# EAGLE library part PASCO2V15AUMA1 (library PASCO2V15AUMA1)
Air Quality Sensors ENVIRONMENTAL SENSING,Carbon Dioxide (CO2) Sensor I2C, PWM, UART Source: Datasheet
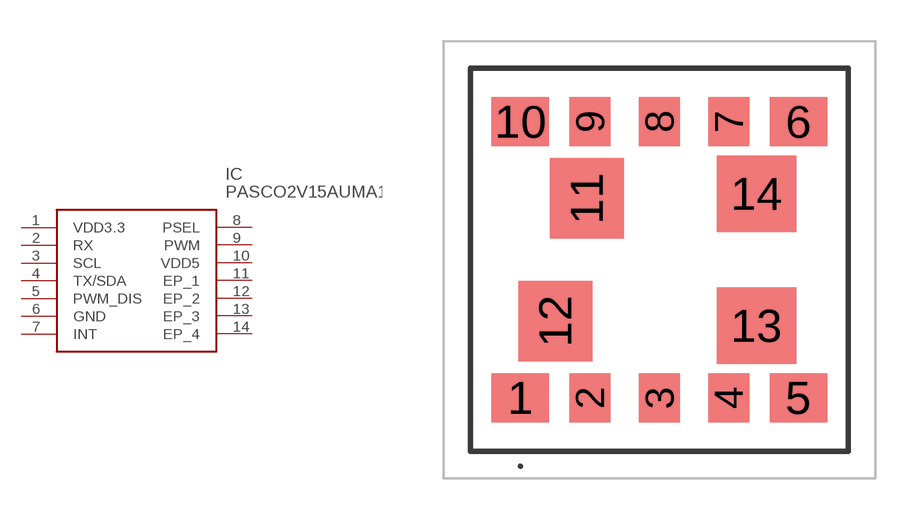
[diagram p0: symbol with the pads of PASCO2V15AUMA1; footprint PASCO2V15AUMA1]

Designator prefix IC

## PASCO2V15AUMA1 (Description: Air Quality Sensors ENVIRONMENTAL SENSING,Carbon Dioxide (CO2) Sensor I2C, PWM, UART; Height: 7.68mm; Manufacturer_Name: Infineon; Manufacturer_Part_Number: PASCO2V15AUMA1; Mouser_Part_Number: 726-PASCO2V15AUMA1; Mouser_Price-Stock: https://www.mouser.co.uk/ProductDetail/Infineon-Technologies/PASCO2V15AUMA1?qs=i8QVZAFTkqQp3OH26KVxRw%3D%3D)  [PASCO2V15AUMA1]
1  VDD3.3
2  RX
3  SCL
4  TX/SDA
5  PWM_DIS
6  GND
7  INT
8  PSEL
9  PWM
10  VDD5
11  EP_1
12  EP_2
13  EP_3
14  EP_4

## Footprint PASCO2V15AUMA1 (pad centres in mm)
LG-MLGA-14_2025-1
smd 2.1 x 1.8: 1 -5.08,-5.05; 5 5.08,-5.05; 6 5.08,5.05; 10 -5.08,5.05
smd 1.5 x 1.8: 2 -2.54,-5.05; 3 0,-5.05; 4 2.54,-5.05; 7 2.54,5.05; 8 0,5.05; 9 -2.54,5.05
smd 2.7 x 2.95: 11 -2.655,2.245; 12 -3.805,-2.245
smd 2.9 x 2.8: 13 3.55,-2.415; 14 3.55,2.415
